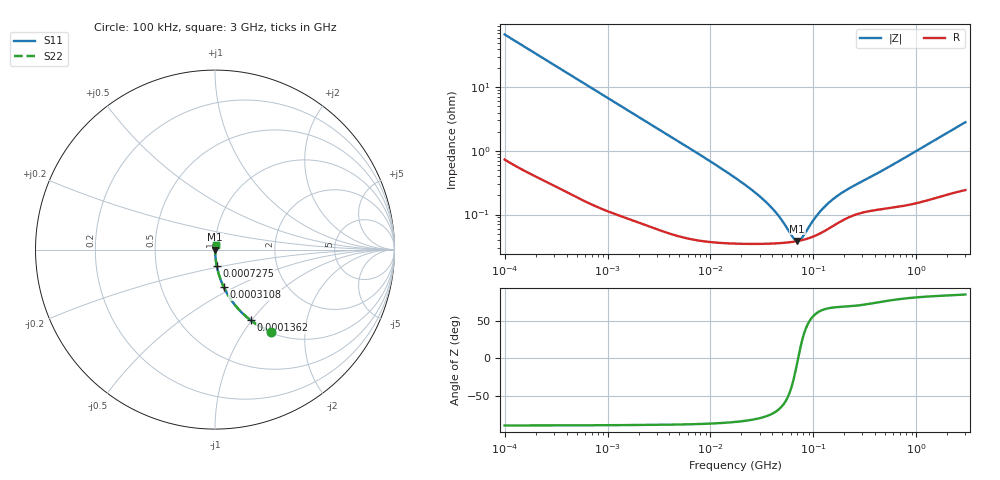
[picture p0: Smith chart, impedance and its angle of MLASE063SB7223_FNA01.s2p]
! MLASE063SB7223_FNA01  S-PARAMETER MODEL  ( Standard Model )
! Model Generated by TAIYO YUDEN Corporation (http://www.ty-top.com)
! Version 1.0
! TAIYO YUDEN Control No. 220601
! Copyright(c) 2013 TAIYO YUDEN CO.,LTD. All Rights Reserved.
! Product Description (link to TY-COMPAS)
! https://ds.yuden.co.jp/TYCOMPAS/or/detail?pn=MLASE063SB7223KFNA01&u=M
! Products Name : Multilayer Ceramic Capacitors
! Characteristics :
!  Capacitance : 0.022 [uF] , Rated Voltage : 16 [V] , TCC : X7R
!  Case Size : 0.6 x 0.3 / 0.024 x 0.012 [mm/inch] , Thickness : 0.3 / 0.012 [mm/inch]
!  (Conditions: Temperature = 25 [degC] , DC Bias Voltage = 0 [V])
! External Node Assignments :
!  1  o---| |---o  2
! GND o---------o GND
! Frequency Range : 100kHz  -  3GHz  [ 401 STEP ]
# MHZ S RI R 50
! Freq[MHz].  S11 Real  S11 Imag  S21 Real  S21 Imag  S12 Real  S12 Imag  S22 Real  S22 Imag
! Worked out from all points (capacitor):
!   401 points, 100 kHz to 3 GHz, reference 50 ohm
!   read as one part in series: C = 23.6 nF near 105.3 kHz
!   lowest |Z| = 38.5 mohm at 69.66 MHz (marker M1)
!   series resonance near 71.09 MHz, so ESL is about 210 pH
!   S11 on the Smith chart (normalised r, x): 100 kHz: 1.01, -1.35; 136.2 kHz: 1.01, -0.99; 310.8 kHz: 1.01, -0.44; 727.5 kHz: 1.00, -0.19; 3 GHz: 1.00, +0.06
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0.1  0.3133 -0.4584  0.6867 0.4584  0.6867 0.4584  0.3133 -0.4584
0.136243  0.1991 -0.3939  0.8009 0.3939  0.8009 0.3939  0.1991 -0.3939
0.200542  0.1047 -0.3003  0.8953 0.3003  0.8953 0.3003  0.1047 -0.3003
0.310802  0.0478 -0.207  0.9522 0.207  0.9522 0.207  0.0478 -0.207
0.562235  0.0161 -0.1189  0.9839 0.1189  0.9839 0.1189  0.0161 -0.1189
0.727522  0.0101 -0.0926  0.9899 0.0926  0.9899 0.0926  0.0101 -0.0926
1.385689  0.00336 -0.0492  0.9966 0.0492  0.9966 0.0492  0.00336 -0.0492
3.161081  0.00105 -0.0218  0.999 0.0218  0.999 0.0218  0.00105 -0.0218
17.7727  0.000362 -0.00367  0.9996 0.00367  0.9996 0.00367  0.000362 -0.00367
27.54426  0.00035 -0.00215  0.9996 0.00215  0.9996 0.00215  0.00035 -0.00215
37.52708  0.00035 -0.00134  0.9996 0.00134  0.9996 0.00134  0.00035 -0.00134
47.32384  0.000356 -0.000821  0.9996 0.000821  0.9996 0.000821  0.000356 -0.000821
62.83488  0.000372 -0.000243  0.9996 0.000243  0.9996 0.000243  0.000372 -0.000243
69.65816  0.000382 -3.98e-05  0.9996 3.98e-05  0.9996 3.98e-05  0.000382 -3.98e-05
73.34282  0.000389 6.15e-05  0.9996 -6.15e-05  0.9996 -6.15e-05  0.000389 6.15e-05
77.22239  0.000396 0.000163  0.9996 -0.000163  0.9996 -0.000163  0.000396 0.000163
97.38194  0.000444 0.000626  0.9996 -0.000626  0.9996 -0.000626  0.000444 0.000626
126.0104  0.000542 0.00116  0.9995 -0.00116  0.9995 -0.00116  0.000542 0.00116
171.6802  0.000731 0.00183  0.9993 -0.00183  0.9993 -0.00183  0.000731 0.00183
227.9507  0.000929 0.00246  0.9991 -0.00246  0.9991 -0.00246  0.000929 0.00246
547.5153  0.00129 0.0055  0.9987 -0.0055  0.9987 -0.0055  0.00129 0.0055
3000  0.0032 0.0279  0.9968 -0.0279  0.9968 -0.0279  0.0032 0.0279
